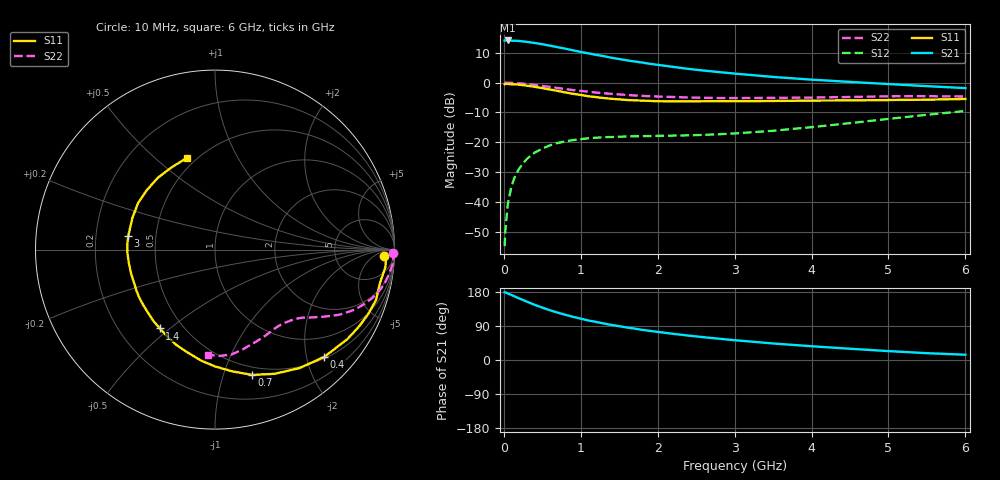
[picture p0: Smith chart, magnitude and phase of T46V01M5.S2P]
! Infineon Technologies  Discrete & RF Semiconductors
! BFR182T
! Si NPN RF Bipolar Junction Transistor in SC75
! VCE = 6 V  IC = 1.5 mA
! Common Emitter S-Parameters:  October  1999
# GHz  S  MA  R  50
!  f  S11  S21  S12  S22
! GHz  MAG  ANG  MAG  ANG  MAG  ANG  MAG  ANG
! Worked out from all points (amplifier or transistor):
!   36 points, 10 MHz to 6 GHz, reference 50 ohm
!   highest |S21| = 14.2 dB at 50 MHz (marker M1)
!   |S21| within 3 dB of that: start of sweep to 843.2 MHz
!   unconditionally stable (mu >= 1): 2.218 GHz to 4.48 GHz
!   at 250 MHz: K = 0.11, MSG = 20.5 dB, |S12| = -27.1 dB
!   at 1.4 GHz: K = 0.68, MSG = 13.3 dB, |S12| = -18.3 dB
!   at 6 GHz: K = 0.83, MSG = 3.8 dB, |S12| = -9.5 dB
!   S11 on the Smith chart (normalised r, x): 10 MHz: 24, -15; 400 MHz: 0.53, -2.34; 700 MHz: 0.42, -1.25; 1.4 GHz: 0.37, -0.46; 3 GHz: 0.34, +0.07; 6 GHz: 0.45, +0.64
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0.01  0.9413 -2.2  5.097 178.5  0.0018 80.9  0.9903 -1.1
0.02  0.9559 -1.1  5.11 178.5  0.0033 79.2  0.9999 -1.0
0.05  0.9541 -5.9  5.119 175.6  0.0089 91.7  0.9952 -2.4
0.1  0.9385 -11.2  5.076 171.5  0.0185 83.6  0.9928 -4.7
0.15  0.9397 -17.5  5.06 166.9  0.0277 80.3  0.9833 -6.9
0.2  0.9261 -22.9  5.011 162.5  0.0361 78.1  0.9746 -9.1
0.3  0.8907 -34.0  4.84 153.9  0.0526 71.1  0.9497 -13.3
0.4  0.8531 -44.5  4.648 145.6  0.0669 65.3  0.9174 -17.1
0.5  0.8109 -54.5  4.423 138.3  0.0781 60.6  0.8831 -20.2
0.6  0.768 -64.3  4.183 131.2  0.0889 55.7  0.849 -23.1
0.7  0.7282 -73.5  3.947 125.0  0.0972 52.2  0.8144 -25.4
0.9  0.6505 -90.1  3.494 113.9  0.1086 46.2  0.752 -29.3
1.1  0.592 -105.2  3.11 104.2  0.1167 41.8  0.7053 -32.1
1.4  0.5362 -125.0  2.622 92.6  0.1223 37.9  0.6502 -35.6
1.6  0.5122 -137.1  2.374 85.7  0.1251 37.0  0.6221 -37.5
1.8  0.5 -147.4  2.176 79.6  0.1269 36.7  0.6 -39.7
2.2  0.4862 -164.0  1.843 69.1  0.1293 38.2  0.5751 -43.7
3  0.4892 171.3  1.423 52.2  0.1406 46.1  0.552 -53.0
3.5  0.493 159.1  1.249 43.6  0.1559 51.7  0.5558 -59.8
4.5  0.504 139.0  1.031 29.7  0.2095 58.4  0.5753 -73.8
5.5  0.5184 117.6  0.875 18.0  0.2895 58.3  0.5931 -87.7
6  0.5334 107.3  0.811 13.9  0.3349 55.8  0.587 -94.0
